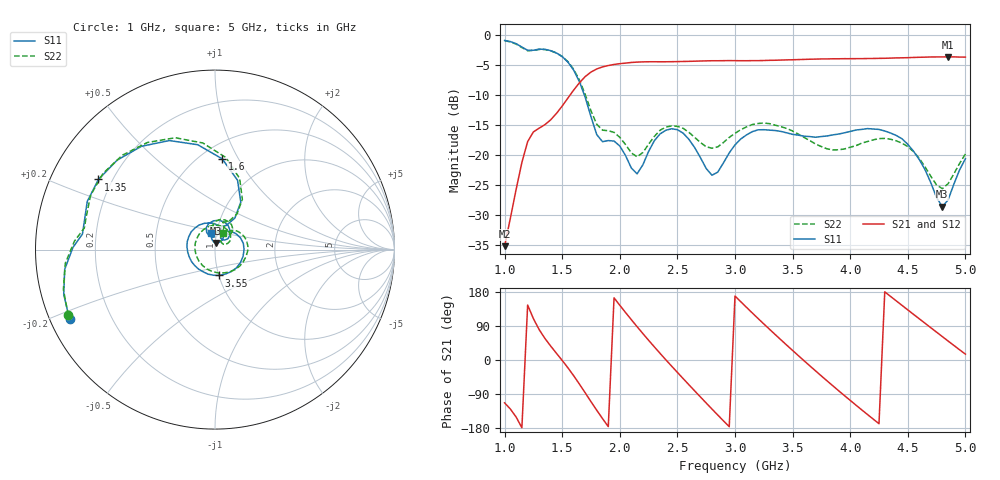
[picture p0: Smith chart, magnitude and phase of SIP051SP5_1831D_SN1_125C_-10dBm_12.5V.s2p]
# GHz  S  dB  R  50
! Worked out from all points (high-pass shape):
!   81 points, 1 GHz to 5 GHz, reference 50 ohm
!   highest |S21| = -3.67 dB at 4.85 GHz (marker M1); lowest = -35.2 dB at 1 GHz (marker M2)
!   |S21| within 3 dB of the highest: 1.719 GHz to end of sweep
!   lowest |S11| = -28.6 dB at 4.8 GHz (marker M3), VSWR 1.08, Z = 50.5 + j3.69 ohm
!   |S11| at or under -10 dB: 1.692 GHz to end of sweep
!   |S22| runs from -25.6 to -1.0 dB; largest |S21 - S12| = 0.0024
!   S11 on the Smith chart (normalised r, x): 1 GHz: 0.06, -0.23; 1.35 GHz: 0.15, +0.27; 1.6 GHz: 0.63, +0.86; 3.55 GHz: 1.00, -0.30; 5 GHz: 0.95, +0.17
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1  -0.93 -154.4  -35.22 -113.1  -35.19 -112.0  -0.96 -155.8
1.2  -2.57 173.3  -17.79 145.0  -17.77 145.1  -2.64 170.6
1.35  -2.41 148.9  -14.96 56.9  -14.96 56.8  -2.44 145.8
1.6  -5.89 85.5  -9.19 -41.7  -9.18 -41.8  -5.74 83.2
1.7  -10.42 61.5  -6.95 -86.7  -6.95 -86.7  -9.95 61.4
1.8  -16.63 65.3  -5.68 -132.7  -5.67 -132.7  -14.91 63.3
1.95  -17.70 80.2  -4.93 164.0  -4.93 164.0  -16.25 72.2
2.15  -23.17 98.2  -4.54 87.9  -4.54 88.0  -20.33 82.5
2.35  -16.50 103.4  -4.48 17.4  -4.48 17.4  -15.89 87.5
2.5  -15.80 71.2  -4.46 -32.8  -4.45 -32.8  -15.25 63.7
2.65  -18.79 44.0  -4.39 -81.5  -4.37 -81.5  -17.09 46.3
2.8  -23.39 54.0  -4.31 -129.4  -4.30 -129.4  -18.89 48.8
3  -18.34 57.4  -4.30 168.8  -4.29 168.8  -16.42 45.4
3.25  -15.80 -0.2  -4.27 95.2  -4.26 95.3  -14.69 6.2
3.55  -16.72 -80.8  -4.12 11.4  -4.11 11.5  -16.55 -56.1
3.7  -17.06 -118.6  -4.04 -28.9  -4.03 -28.9  -18.20 -97.3
4  -16.10 174.6  -3.97 -106.5  -3.97 -106.5  -18.73 162.4
4.35  -16.36 102.1  -3.87 167.9  -3.89 167.8  -17.39 71.2
4.6  -20.79 58.0  -3.73 108.6  -3.73 108.5  -20.58 29.1
4.8  -28.64 80.5  -3.67 61.7  -3.68 61.7  -25.63 43.9
4.85  -27.50 99.3  -3.67 50.0  -3.67 50.1  -24.81 56.7
5  -20.66 102.2  -3.71 15.5  -3.71 15.5  -19.86 63.2
